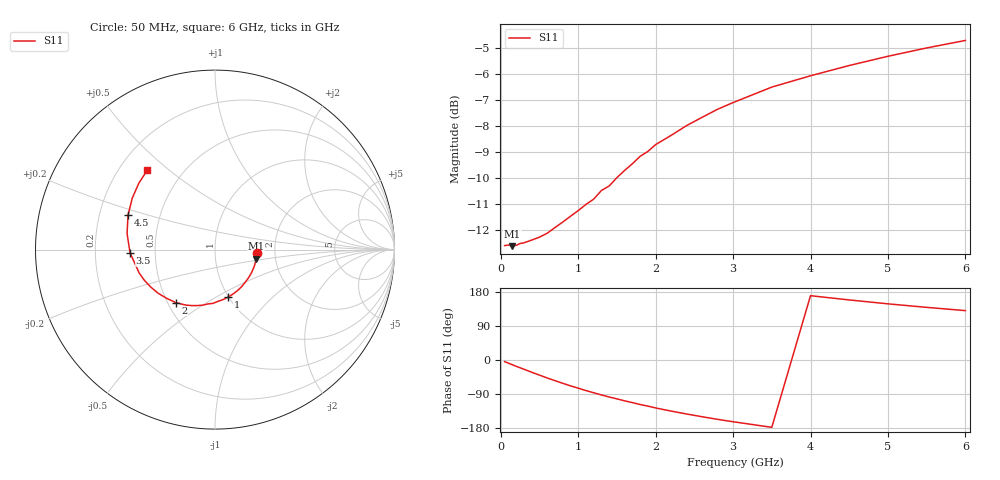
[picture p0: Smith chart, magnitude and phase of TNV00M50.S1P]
! SIEMENS Discrete & RF Semiconductors
! BAS70-07W
! Si Schottky Diode in SOT343
! IF = 0.5 mA
! S-Parameters:  February  1997
# GHz  S  MA  R  50
!  f  S11
! GHz  MAG  ANG
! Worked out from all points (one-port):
!   34 points, 50 MHz to 6 GHz, reference 50 ohm
!   lowest |S11| = -12.6 dB at 150 MHz (marker M1), VSWR 1.61, Z = 79.1 - j8.49 ohm
!   |S11| at or under -10 dB: start of sweep to 1.491 GHz
!   S11 on the Smith chart (normalised r, x): 50 MHz: 1.61, -0.06; 1 GHz: 1.00, -0.57; 2 GHz: 0.55, -0.38; 3.5 GHz: 0.36, -0.02; 4.5 GHz: 0.33, +0.17; 6 GHz: 0.32, +0.42
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0.05  0.2349 -4.3
0.15  0.2344 -12.5
0.25  0.2371 -20.5
0.4  0.2408 -32.3
0.6  0.2481 -47.4
0.8  0.2606 -61.4
1  0.2742 -74.3
1.1  0.2819 -80.7
1.2  0.2885 -86.4
1.3  0.2998 -92.2
1.4  0.3058 -97.6
1.5  0.3173 -102.6
1.6  0.3276 -107.8
1.7  0.3375 -112.4
1.8  0.3487 -117.5
1.9  0.3563 -121.7
2  0.3672 -126.5
2.2  0.3825 -134.8
2.4  0.3994 -142.5
2.6  0.4143 -149.7
2.8  0.4293 -156.6
3  0.4422 -162.9
3.5  0.4735 -177.7
4  0.4978 169.7
4.5  0.521 158.5
5  0.5427 148.2
5.5  0.5631 138.9
6  0.582 130.3
